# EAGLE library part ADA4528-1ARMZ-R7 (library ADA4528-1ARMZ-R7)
Check availability
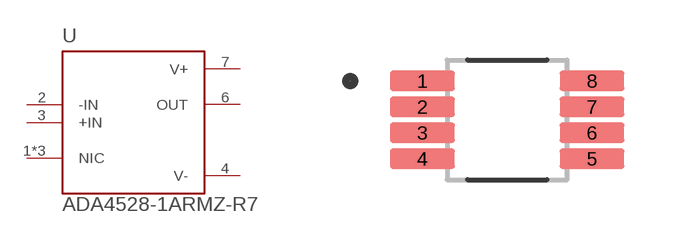
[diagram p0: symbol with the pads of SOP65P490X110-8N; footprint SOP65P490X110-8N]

Designator prefix U

## ADA4528-1ARMZ-R7 (Availability: In Stock; Check_prices: https://www.snapeda.com/parts/ADA4528-1ARMZ-R7/Analog+Devices/view-part/?ref=eda; Description: Precision, Ultralow Noise, RRIO, Zero-Drift Single Op Amp; MF: Analog Devices; MP: ADA4528-1ARMZ-R7; Package: MSOP-8 Analog Devices; Price: None; SnapEDA_Link: https://www.snapeda.com/parts/ADA4528-1ARMZ-R7/Analog+Devices/view-part/?ref=snap)  [SOP65P490X110-8N]
1  NIC  nc
2  -IN  in
3  +IN  in
4  V-  pwr
5  NIC  nc
6  OUT  out
7  V+  pwr
8  NIC  nc

## Footprint SOP65P490X110-8N (pad centres in mm)
smd 1.62 x 0.5: 1 -2.12,0.975; 2 -2.12,0.325; 3 -2.12,-0.325; 4 -2.12,-0.975; 5 2.12,-0.975; 6 2.12,-0.325; 7 2.12,0.325; 8 2.12,0.975

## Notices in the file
This work is licensed under a Creative Commons Attribution-ShareAlike 4.0 International License (CC BY-SA) with Design Exception 1.0
